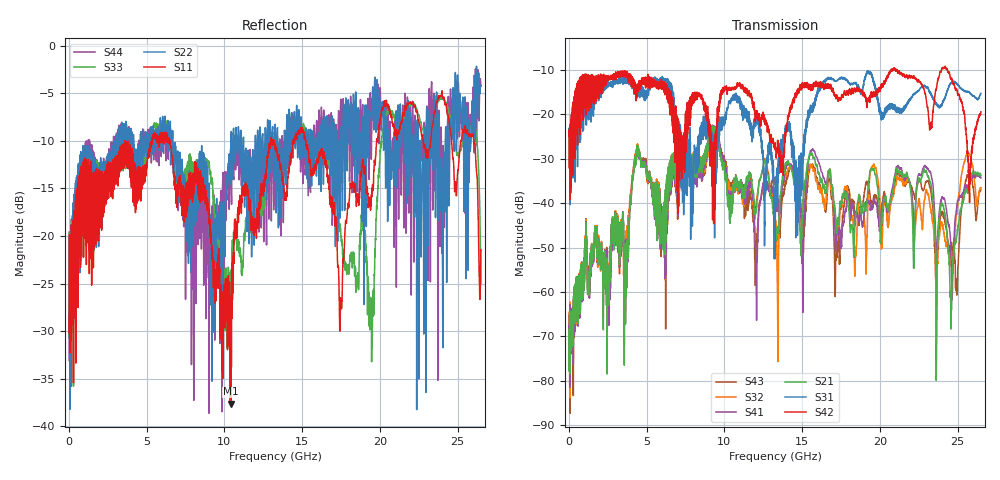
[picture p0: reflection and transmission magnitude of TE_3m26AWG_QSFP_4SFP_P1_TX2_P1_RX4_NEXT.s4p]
!Agilent Technologies,N5222A,MY51421691,A.10.00.00
!Agilent N5222A: A.10.00.00
!Date: Friday, January 30, 2015 12:34:51
!Correction: S11(Full 4 Port(1,2,3,4))
!S12(Full 4 Port(1,2,3,4))
!S13(Full 4 Port(1,2,3,4))
!S14(Full 4 Port(1,2,3,4))
!S21(Full 4 Port(1,2,3,4))
!S22(Full 4 Port(1,2,3,4))
!S23(Full 4 Port(1,2,3,4))
!S24(Full 4 Port(1,2,3,4))
!S31(Full 4 Port(1,2,3,4))
!S32(Full 4 Port(1,2,3,4))
!S33(Full 4 Port(1,2,3,4))
!S34(Full 4 Port(1,2,3,4))
!S41(Full 4 Port(1,2,3,4))
!S42(Full 4 Port(1,2,3,4))
!S43(Full 4 Port(1,2,3,4))
!S44(Full 4 Port(1,2,3,4))
!S4P File: Measurements: <S11,S12,S13,S14>,
!<S21,S22,S23,S24>,
!<S31,S32,S33,S34>,
!<S41,S42,S43,S44>:
# Hz S  dB  R 50.0
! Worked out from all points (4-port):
!   2650 points, 10 MHz to 26.5 GHz, reference 50 ohm
!   strongest paths, dB at 10 MHz, 6.63 GHz, 13.26 GHz, 19.88 GHz, 26.5 GHz:
!     S42: -25.0, -19.3, -26.9, -14.9, -19.4
!     S31: -24.7, -15.5, -42.5, -17.4, -15.3
!     S21: -68.4, -29.0, -46.7, -37.1, -33.8
!     S41: -65.3, -29.4, -39.3, -42.9, -34.3
!     S32: -64.6, -29.1, -44.2, -34.9, -36.5
!     S43: -67.6, -29.6, -35.8, -40.6, -36.9
!   lowest |S11| = -37.6 dB at 10.42 GHz (marker M1), VSWR 1.03, Z = 48.8 + j0.468 ohm
!   |S11| at or under -10 dB: start of sweep to 3.58 GHz; 6.485 GHz to 12.98 GHz (6.494 GHz wide, 66.7 % of centre); 15.24 GHz to 19.79 GHz (4.547 GHz wide, 26 % of centre)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
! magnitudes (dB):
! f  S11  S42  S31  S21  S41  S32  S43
! 10 MHz  -19.9  -25.0  -24.7  -68.4  -65.3  -64.6  -67.6
! 4.4 GHz  -15.1  -15.4  -15.9  -28.8  -29.0  -28.5  -28.8
! 10.42 GHz  -37.6  -14.5  -17.0  -38.3  -37.3  -36.5  -35.3
! 13.3 GHz  -11.1  -27.5  -36.3  -46.5  -39.6  -43.9  -35.7
! 22.91 GHz  -10.6  -15.3  -13.6  -32.9  -31.5  -38.4  -35.8
! 24.58 GHz  -9.4  -11.9  -12.9  -68.4  -52.1  -53.1  -49.1
! 26.5 GHz  -21.4  -19.4  -15.3  -33.8  -34.3  -36.5  -36.9
